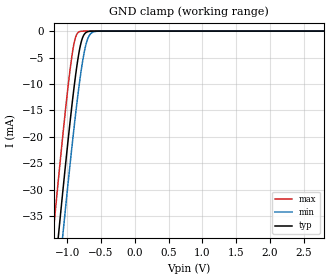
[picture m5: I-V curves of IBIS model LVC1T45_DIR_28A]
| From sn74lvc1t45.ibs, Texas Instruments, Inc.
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[Model]   LVC1T45_DIR_28A
Model_type  Input
Vinl=0.7
Vinh=1.7
| variable   typ   min   max
C_comp   3.10pF   2.52pF   4.22pF
[Temperature Range]   40   100   -40
| Ambient temperature   25   85   -40
[Voltage range]   2.8   2.8   2.8
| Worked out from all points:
|   GND clamp passes 1 mA (typ) near -0.77 V on its own axis
[GND Clamp]
| LVC1T45_DIR_28A
|   Voltage   I(typ)   I(min)   I(max)
-5.5V     -655.2mA   -662.2mA   -646.6mA
-1.205V   -48.27mA   -56.56mA   -37.63mA
-1.13V    -38.42mA   -46.71mA   -27.77mA
-1.07V    -30.71mA   -38.96mA   -20.13mA
-1.055V   -28.82mA   -37.05mA   -18.27mA
-955mV    -16.68mA   -24.66mA   -6.874mA
-885mV    -9.098mA   -16.55mA   -1.486mA
-825mV    -3.922mA   -10.26mA   -137.1uA
-780mV    -1.472mA   -6.227mA   -17.15uA
-710mV    -173.7uA   -1.918mA   -639nA
-645mV    -18.49uA   -387.7uA   -29.98nA
2.8V      5.309pA    7.956pA    5.085pA
